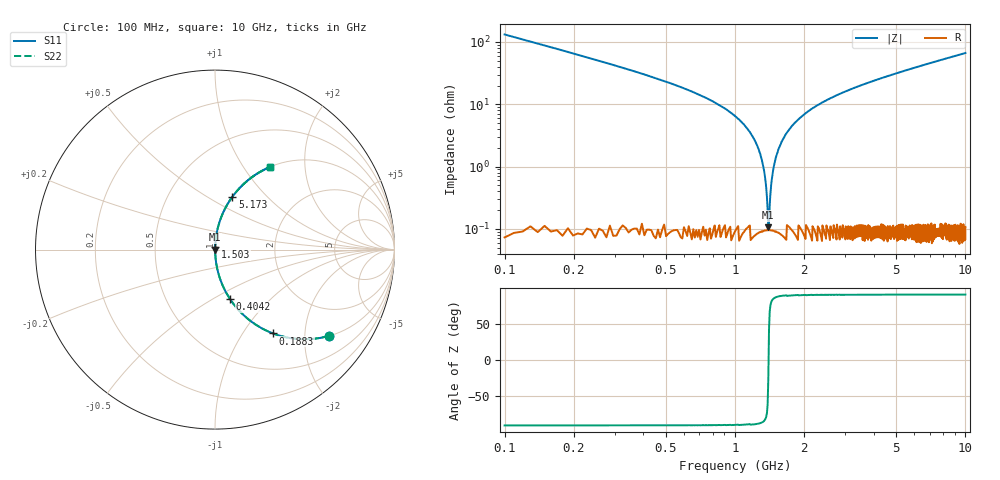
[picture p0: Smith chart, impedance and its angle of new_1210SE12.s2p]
!	AVX	Thin	Film	Operation	Date:	April 2007
!	Description:	Accu-P®	"Series,"	Thin	"Film,"	"SMD,"	RF	Capacitor
!	Part	Number:	12101J120FBT
!	100	MHz	-	5.05	GHz
!	Serial	Measurements
#	MHZ	S	MA	R	50
!	S11	S21	S12	S22
!	dB	Phase	dB	Phase	dB	Phase	dB	Phase
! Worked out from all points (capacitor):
!   1010 points, 100 MHz to 10 GHz, reference 50 ohm
!   read as one part in series: C = 12 pF near 149.1 MHz
!   lowest |Z| = 105 mohm at 1.395 GHz (marker M1)
!   series resonance near 1.399 GHz, so ESL is about 1.1 nH
!   S11 on the Smith chart (normalised r, x): 100 MHz: 1.00, -2.64; 188.3 MHz: 1.00, -1.38; 404.2 MHz: 1.00, -0.60; 1.503 GHz: 1.00, +0.03; 5.173 GHz: 1.00, +0.65; 10 GHz: 1.00, +1.33
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100  0.797 -37.1  0.604 52.8  0.604 52.8  0.797 -37.1
188.305  0.568 -55.3  0.822 34.6  0.822 34.6  0.568 -55.3
276.611  0.418 -65.2  0.908 24.7  0.908 24.7  0.418 -65.2
404.163  0.288 -73.1  0.957 16.7  0.957 16.7  0.288 -73.1
914.371  0.083 -84.6  0.996 4.7  0.996 4.7  0.083 -84.6
1140.04  0.039 -86.4  0.998 2.2  0.998 2.2  0.039 -86.4
1277.403  0.017 -86.0  0.999 1.0  0.999 1.0  0.017 -86.0
1316.65  0.011 -84.8  0.999 0.7  0.999 0.7  0.011 -84.8
1365.709  0.00459 -78.4  0.999 0.3  0.999 0.3  0.00459 -78.4
1395.144  0.00101 -27.0  0.999 0.0  0.999 0.0  0.00101 -27.0
1434.39  0.00488 79.1  0.999 -0.3  0.999 -0.3  0.00488 79.1
1473.637  0.00996 84.2  0.999 -0.6  0.999 -0.6  0.00996 84.2
1503.072  0.014 85.5  0.999 -0.8  0.999 -0.8  0.014 85.5
1601.189  0.026 86.5  0.999 -1.5  0.999 -1.5  0.026 86.5
1758.176  0.044 86.3  0.998 -2.5  0.998 -2.5  0.044 86.3
2337.066  0.101 83.7  0.994 -5.8  0.994 -5.8  0.101 83.7
3406.541  0.188 78.9  0.981 -10.9  0.981 -10.9  0.188 78.9
5054.906  0.302 72.3  0.953 -17.6  0.953 -17.6  0.302 72.3
5172.646  0.309 71.8  0.95 -18.0  0.95 -18.0  0.309 71.8
6703.271  0.398 66.4  0.916 -23.5  0.916 -23.5  0.398 66.4
8351.635  0.482 61.1  0.875 -28.8  0.875 -28.8  0.482 61.1
10000  0.553 56.3  0.832 -33.6  0.832 -33.6  0.553 56.3
